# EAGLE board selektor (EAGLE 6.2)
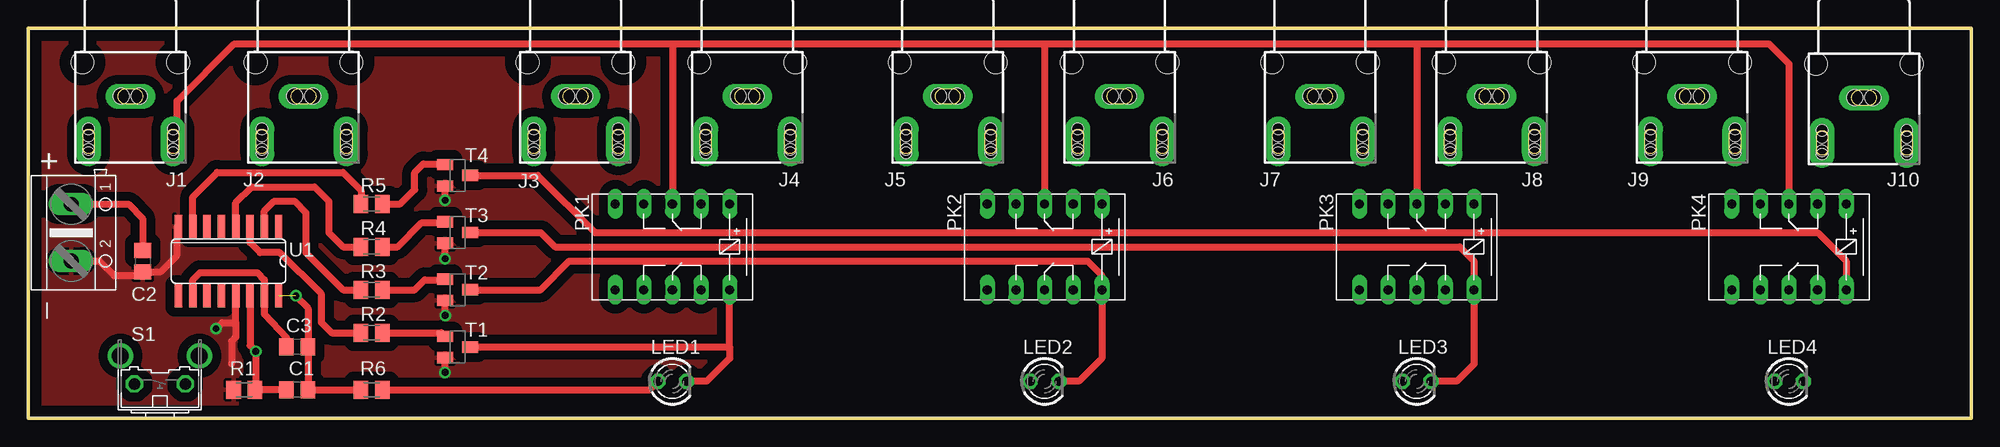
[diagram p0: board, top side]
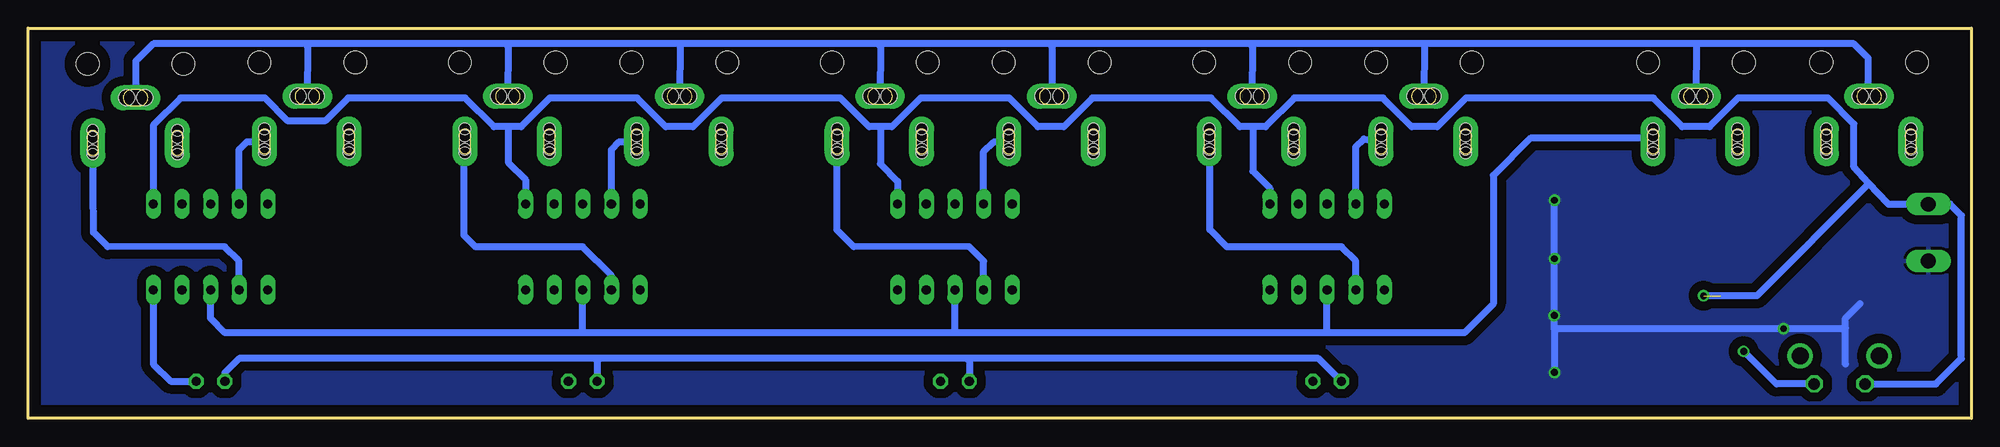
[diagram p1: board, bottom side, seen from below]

Size 172.39 x 34.66 mm. Coordinates in mm from the lower left corner, seen from the top.
Outline: 0,0 172.39,0 172.39,34.66 0,34.66 0,0
Copper layers (1*16): Top 0.035mm / dielectric 1.5mm / Bottom 0.035mm
Design rules: minimum track width 10mil, minimum drill 24mil, track to track 8mil, track to pad 8mil, pad to pad 8mil, via to via 8mil, smd to smd 8mil, copper to edge 40mil, drill to drill 8mil, minimum pad ring 10mil, minimum via ring 8mil, stop-mask expansion 4mil, vias tented up to drill 0mil, thermal gap 10mil

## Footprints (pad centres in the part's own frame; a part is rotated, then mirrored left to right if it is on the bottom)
C0805 = smd 1.3 x 1.5: 1 -0.95,0; 2 0.95,0
WBTOR1 = drill 1.4 pad 2.2 long: S 5,6 | drill 1 pad 2.2 long: T 8.8,2; T1 1.3,2 | hole 2: 0.75,9; 9.25,9 | hole 1: 1.3,2.5; 1.3,1.3; 1.3,1; 1.3,3.1; 8.8,3.1; 8.8,2.5; 8.8,1.3; 8.8,1 | hole 1.4: 4.2,6; 5.8,6
LED3MM = drill 0.813 octagon: A -1.27,0; K 1.27,0
G6H2-100 = drill 0.813 long: 1 -5.08,-3.81; 5 5.08,-3.81; 6 5.08,3.81; 10 -5.08,3.81; O1 -2.54,-3.81; O2 -2.54,3.81; P1 0,-3.81; P2 0,3.81; S1 2.54,-3.81; S2 2.54,3.81
M0805 = smd 1.3 x 1.6: 1 -0.95,0; 2 0.95,0
B3F-31XX = drill 1.016 octagon: 1 -2.261,-1.245; 2 2.261,-1.245 | drill 1.499 pad 2.159: 3 -3.505,1.245; 4 3.505,1.245
SOT23-BEC = smd 1 x 1.4: B -0.95,-1.1; C 0,1.1; E 0.95,-1.1
SO16 = smd 0.66 x 2.032: 1 -4.445,-3.073; 2 -3.175,-3.073; 3 -1.905,-3.073; 4 -0.635,-3.073; 5 0.635,-3.073; 6 1.905,-3.073; 7 3.175,-3.073; 8 4.445,-3.073; 9 4.445,3.073; 10 3.175,3.073; 11 1.905,3.073; 12 0.635,3.073; 13 -0.635,3.073; 14 -1.905,3.073; 15 -3.175,3.073; 16 -4.445,3.073
AK500/2 = drill 1.321 long: 1 -2.515,0; 2 2.515,0

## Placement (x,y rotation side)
C1  100nF  [C0805]  23.88,2.54 180 top
C2  100nF  [C0805]  10.16,13.97 270 top
C3  10nF  [C0805]  23.88,6.35 180 top
J1  OUT  [WBTOR1]  4.06,22.61 0 top
J2  [WBTOR1]  19.43,22.61 0 top
J3  IN1  [WBTOR1]  43.56,22.61 0 top
J4  [WBTOR1]  58.8,22.61 0 top
J5  IN2  [WBTOR1]  76.58,22.61 0 top
J6  [WBTOR1]  91.82,22.61 0 top
J7  IN3  [WBTOR1]  109.6,22.61 0 top
J8  [WBTOR1]  124.84,22.61 0 top
J9  IN4  [WBTOR1]  142.62,22.61 0 top
J10  [WBTOR1]  157.86,22.48 0 top
LED1  [LED3MM]  57.15,3.3 0 top
LED2  [LED3MM]  90.17,3.3 0 top
LED3  [LED3MM]  123.19,3.3 0 top
LED4  [LED3MM]  156.21,3.3 0 top
PK1  [G6H2-100]  57.15,15.24 180 top
PK2  [G6H2-100]  90.17,15.24 180 top
PK3  [G6H2-100]  123.19,15.24 180 top
PK4  [G6H2-100]  156.21,15.24 180 top
R1  10k  [M0805]  19.18,2.54 0 top
R2  [M0805]  30.48,7.62 180 top
R3  [M0805]  30.48,11.43 180 top
R4  [M0805]  30.48,15.24 180 top
R5  [M0805]  30.48,19.05 180 top
R6  [M0805]  30.48,2.54 180 top
S1  [B3F-31XX]  11.68,4.32 0 top
T1  BC847  [SOT23-BEC]  38.1,6.35 270 top
T2  BC847  [SOT23-BEC]  38.1,11.43 270 top
T3  BC847  [SOT23-BEC]  38.1,16.51 270 top
T4  BC847  [SOT23-BEC]  38.1,21.59 270 top
U1  4017D  [SO16]  17.78,13.97 180 top
X11  [AK500/2]  3.81,16.51 270 top

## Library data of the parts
C1-C3 R1-R6 = rcl
J1-J10 = con-lumberg; MPN: WBTOR 1 BLACK; OC_FARNELL: 1200146; OC_NEWARK: 98K2588
LED1-LED4 = led
PK1-PK4 = relay
S1 = switch-omron
T1-T4 = transistor
U1 = 40xx
X11 = con-ptr500

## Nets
GND: C2.2 R1.1 T1.E T2.E T3.E T4.E U1.8 U1.13 X11.2
GND2: J1.S J2.S J3.S J4.S J5.S J6.S J7.S J8.S J9.S J10.S
N$1: C3.2 U1.10 U1.15
N$2: R2.2 U1.3
N$4: R3.2 U1.2
N$5: R4.2 U1.4
N$6: R5.2 U1.7
N$7: R2.1 T1.B
N$8: R5.1 T4.B
N$9: R3.1 T2.B
N$10: R4.1 T3.B
N$11: LED4.K PK4.10 T4.C
N$12: LED3.K PK3.10 T3.C
N$13: LED2.K PK2.10 T2.C
N$14: LED1.K PK1.10 T1.C
N$15: LED1.A LED2.A LED3.A LED4.A R6.1
N$16: J1.T PK1.P1 PK2.P1 PK3.P1 PK4.P1
N$17: J2.T PK1.P2 PK2.P2 PK3.P2 PK4.P2
N$18: J3.T PK1.S1
N$19: J4.T PK1.S2
N$20: J6.T PK2.S2
N$21: J5.T PK2.S1
N$22: J7.T PK3.S1
N$23: J8.T PK3.S2
N$24: J9.T PK4.S1
N$25: J10.T PK4.S2
N$26: C1.2 R1.2 S1.2 U1.14
VCC: C1.1 C2.1 C3.1 PK1.1 PK2.1 PK3.1 PK4.1 R6.2 S1.1 U1.16 X11.1

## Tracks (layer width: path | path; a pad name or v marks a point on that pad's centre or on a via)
GND  (via drill 0.6)
  Top 0.61: X11.2 6.33,13.99 7.62,12.7 9.84,12.7 C2.2 11.75,13.02 13.21,14.48 13.21,16.92 U1.8 | 18.41,8.51 18.41,7.24 18.03,6.86 18.03,4.89 | T4.E 37,19.4 v36.98,19.38 | v36.98,14.2 36.98,15.54 T3.E | T2.E v37,9.15 v37.01,9.14 | v36.98,4.09 36.98,5.38 T1.E | 18.41,8.51 U1.13 | 18.41,8.51 17.2,8.51 v16.66,7.98
  Bottom 0.61: 9.88,10.19 11.18,8.89 11.18,8.03 | 11.18,4.83 11.18,8.03 | v36.98,19.38 v36.98,14.2 37.01,14.17 v37.01,9.14 | 37,7.98 37,4.11 v36.98,4.09 | 37,7.98 v37,9.15 | 37,7.98 v16.66,7.98 11.23,7.98 11.18,8.03
  pour Bottom (isolate 0.813): -0.25,35.94 172.47,35.94 172.72,-0.51 0,-0.51
  pour Top (isolate 0.813): -0.38,36.07 172.59,35.81 172.97,-0.51 -0.25,-0.51
GND2
  Bottom 0.61: J10.S 162.83,31.73 161.29,33.27 147.83,33.27 | 130.05,33.27 147.83,33.27 | J9.S 147.59,33.04 147.83,33.27 | J8.S 129.81,33.04 130.05,33.27 | 24.38,33.27 10.41,33.27 9.14,32 9.14,28.85 J1.S | 24.38,33.27 48.51,33.27 | 48.51,33.27 64.01,33.27 | 64.01,33.27 81.79,33.27 | 81.79,33.27 97.03,33.27 | 97.03,33.27 114.55,33.27 | 114.55,33.27 130.05,33.27 | J2.S 24.4,33.26 24.38,33.27 | J3.S 48.53,33.26 48.51,33.27 | J4.S 63.77,33.04 64.01,33.27 | J5.S 81.55,33.04 81.79,33.27 | J6.S 96.79,33.04 97.03,33.27 | J7.S 114.57,33.26 114.55,33.27
N$1
  Top 0.61: U1.10 14.61,12.32 15.24,12.95 20.32,12.95 20.96,12.32 U1.15 20.96,9.27 22.93,7.17 C3.2
N$2
  Top 0.61: U1.3 19.69,15.62 20.57,14.73 22.33,14.73 26.04,11.05 26.04,8.51 26.92,7.62 R2.2
N$4
  Top 0.61: U1.2 20.96,18.41 21.84,19.3 23.62,19.3 24.64,18.29 24.64,14.73 27.94,11.43 R3.2
N$5
  Top 0.61: U1.4 18.41,19.18 19.81,20.57 25.4,20.57 26.67,19.3 26.67,16.51 27.94,15.24 R4.2
N$6
  Top 0.61: R5.2 29.53,20.25 27.94,21.84 16.76,21.84 14.61,19.69 U1.7
N$7
  Top 0.61: R2.1 36.68,7.62 T1.B
N$8
  Top 0.61: R5.1 33.02,19.05 34.29,20.32 34.29,21.84 35.05,22.61 36.55,22.61 T4.B
N$9
  Top 0.61: R3.1 34.29,11.43 35.18,12.32 36.93,12.32 T2.B
N$10
  Top 0.61: R4.1 32.77,15.24 34.92,17.4 36.81,17.4 T3.B
N$11
  Top 0.61: T4.C 45.21,21.59 50.29,16.51 158.75,16.51 161.29,13.97 PK4.10
  Bottom 0.61: LED4.K 159.77,3.3 161.29,4.83 PK4.10
N$12
  Top 0.61: T3.C 45.47,16.51 46.74,15.24 127,15.24 128.27,13.97 PK3.10 128.27,4.83 126.75,3.3 LED3.K
N$13
  Top 0.61: T2.C 45.47,11.43 48.01,13.97 93.98,13.97 95.25,12.7 PK2.10 95.25,5.33 93.22,3.3 LED2.K
N$14
  Top 0.61: 62.23,6.35 62.23,5.33 60.2,3.3 LED1.K | 62.23,6.35 PK1.10 | T1.C 62.23,6.35
N$15
  Top 0.61: R6.1 55.12,2.54 LED1.A
  Bottom 0.61: LED4.A 154.94,4.06 153.67,5.33 121.67,5.33 | 89.15,5.33 57.91,5.33 LED1.A | 89.15,5.33 121.67,5.33 | LED2.A 88.9,5.08 89.15,5.33 | LED3.A 121.92,5.08 121.67,5.33
N$16
  Top 0.61: 57.15,33.27 PK1.P1 | 57.15,33.27 18.29,33.27 13.21,28.19 13.21,24.88 J1.T | PK4.P1 156.21,31.5 154.43,33.27 123.19,33.27 | 57.15,33.27 90.17,33.27 | 90.17,33.27 123.19,33.27 | 123.19,33.27 PK3.P1 | 90.17,33.27 PK2.P1
N$17
  Bottom 0.61: 57.15,7.62 90.17,7.62 | 90.17,7.62 123.19,7.62 | 123.19,7.62 154.94,7.62 156.21,8.89 PK4.P2 | 57.15,7.62 PK1.P2 | 90.17,7.62 PK2.P2 | 123.19,7.62 PK3.P2 | 57.15,7.62 44.96,7.62 42.42,10.16 42.42,21.59 39.12,24.89 28.46,24.89 J2.T
N$18
  Bottom 0.61: 54.83,19.27 PK1.S1 54.61,24.13 53.91,24.83 J3.T
N$19
  Bottom 0.61: PK1.S2 54.61,13.97 55.88,15.24 66.04,15.24 67.56,16.76 67.56,23.49 67.63,24.7 J4.T
N$20
  Bottom 0.61: J6.T 100.65,16.76 99.16,15.27 88.9,15.24 87.63,13.97 PK2.S2
N$21
  Bottom 0.61: PK2.S1 87.63,23.72 86.74,24.54 86.68,24.58 J5.T
N$22
  Bottom 0.61: J7.T 119.95,24.58 120.65,23.88 120.62,19.52 PK3.S1
N$23
  Bottom 0.61: PK3.S2 120.65,12.7 123.19,15.24 132.72,15.24 133.73,16.26 133.73,22.83 J8.T
N$24
  Bottom 0.61: J9.T 152.97,24.58 153.67,23.88 PK4.S1
N$25
  Bottom 0.61: J10.T 166.59,16.5 165.35,15.27 154.94,15.24 153.67,13.97 PK4.S2
N$26  (via drill 0.6)
  Top 0.61: C1.2 R1.2 20.19,2.61 20.19,5.46 v20.19,5.97 19.69,6.48 U1.14
  Bottom 0.61: S1.2 17.3,3.07 v20.19,5.97
VCC  (via drill 0.6)  (1 unrouted)
  Top 0.508: 24.77,9.91 24.83,9.78
  Top 0.61: C3.1 24.83,6.42 | v23.75,10.9 24.77,9.91 | 24.83,9.78 C3.1 | C3.1 C1.1 R6.2 | X11.1 8.92,19.02 10.16,17.78 C2.1
  Bottom 0.61: PK4.1 161.29,26.04 158.88,28.45 151.38,28.45 149.35,26.42 146.05,26.42 144.02,28.45 133.6,28.45 131.06,25.91 129.79,25.91 | 129.79,25.91 128.65,25.91 126.11,28.45 118.36,28.45 115.82,25.91 113.41,25.91 110.87,28.45 100.33,28.45 97.79,25.91 96.77,25.91 | 63.75,25.91 64.9,25.91 67.44,28.45 77.98,28.45 80.52,25.91 82.8,25.91 85.34,28.45 93.22,28.45 95.76,25.91 96.77,25.91 | 9.11,20.87 7.37,19.02 X11.1 3.79,19.05 1.91,19.05 0.89,18.03 0.89,5.33 3.15,3.07 S1.1 | 9.11,20.87 10.41,22.33 10.41,26.16 12.7,28.45 20.7,28.45 23.24,25.91 25.65,25.91 28.19,28.45 44.83,28.45 47.37,25.91 49.66,25.91 52.2,28.45 60.07,28.45 62.61,25.91 63.75,25.91 | 129.79,25.91 129.79,22.73 128.27,21.21 PK3.1 | PK2.1 95.25,21.06 96.77,22.61 96.77,25.91 | 63.75,25.91 63.75,21.97 62.23,20.45 PK1.1 | v23.75,10.9 19.02,10.9 9.11,20.87

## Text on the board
tNames: + | _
